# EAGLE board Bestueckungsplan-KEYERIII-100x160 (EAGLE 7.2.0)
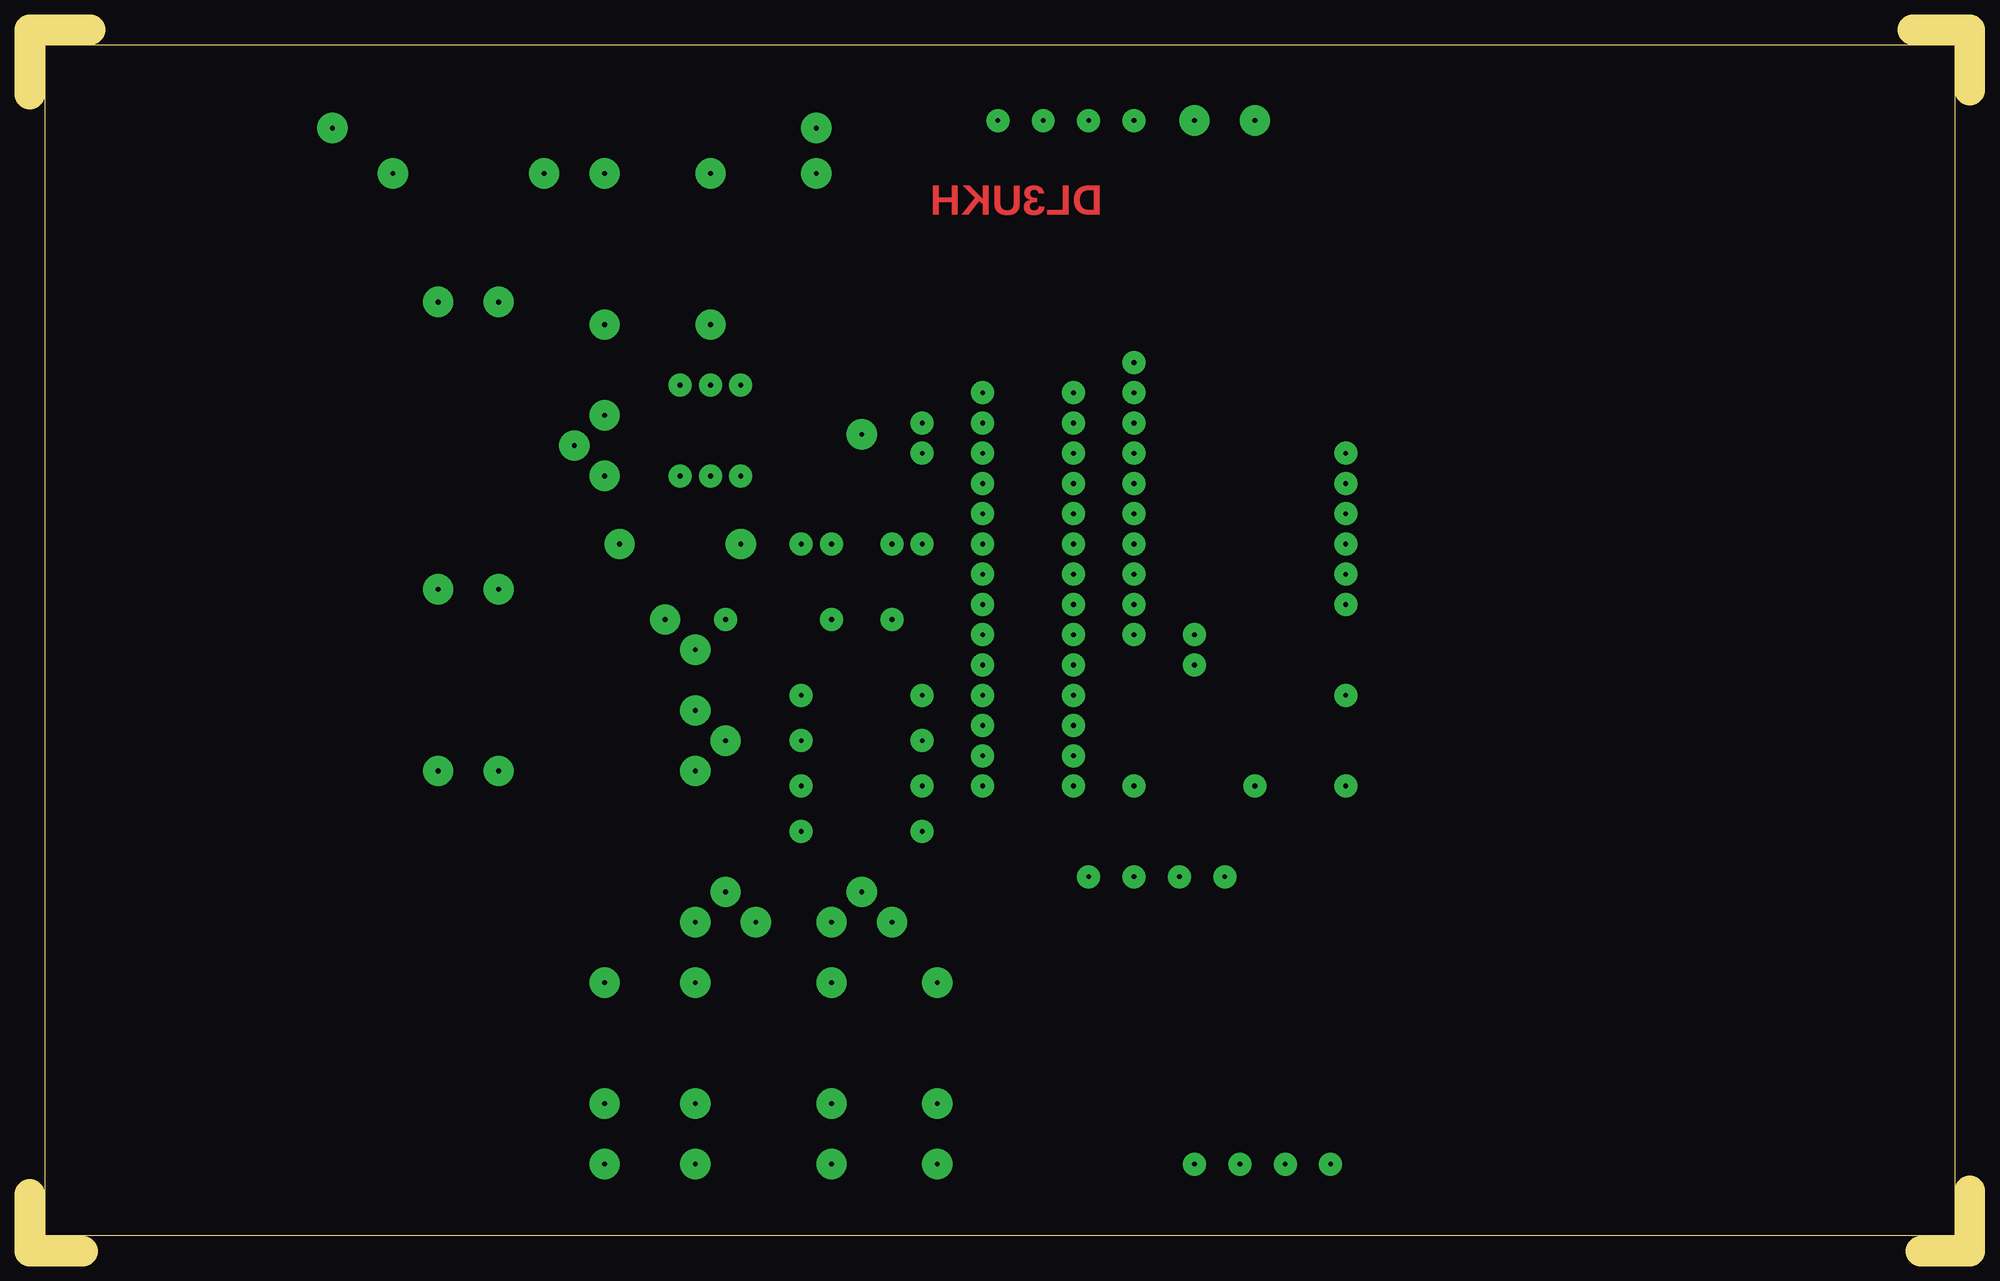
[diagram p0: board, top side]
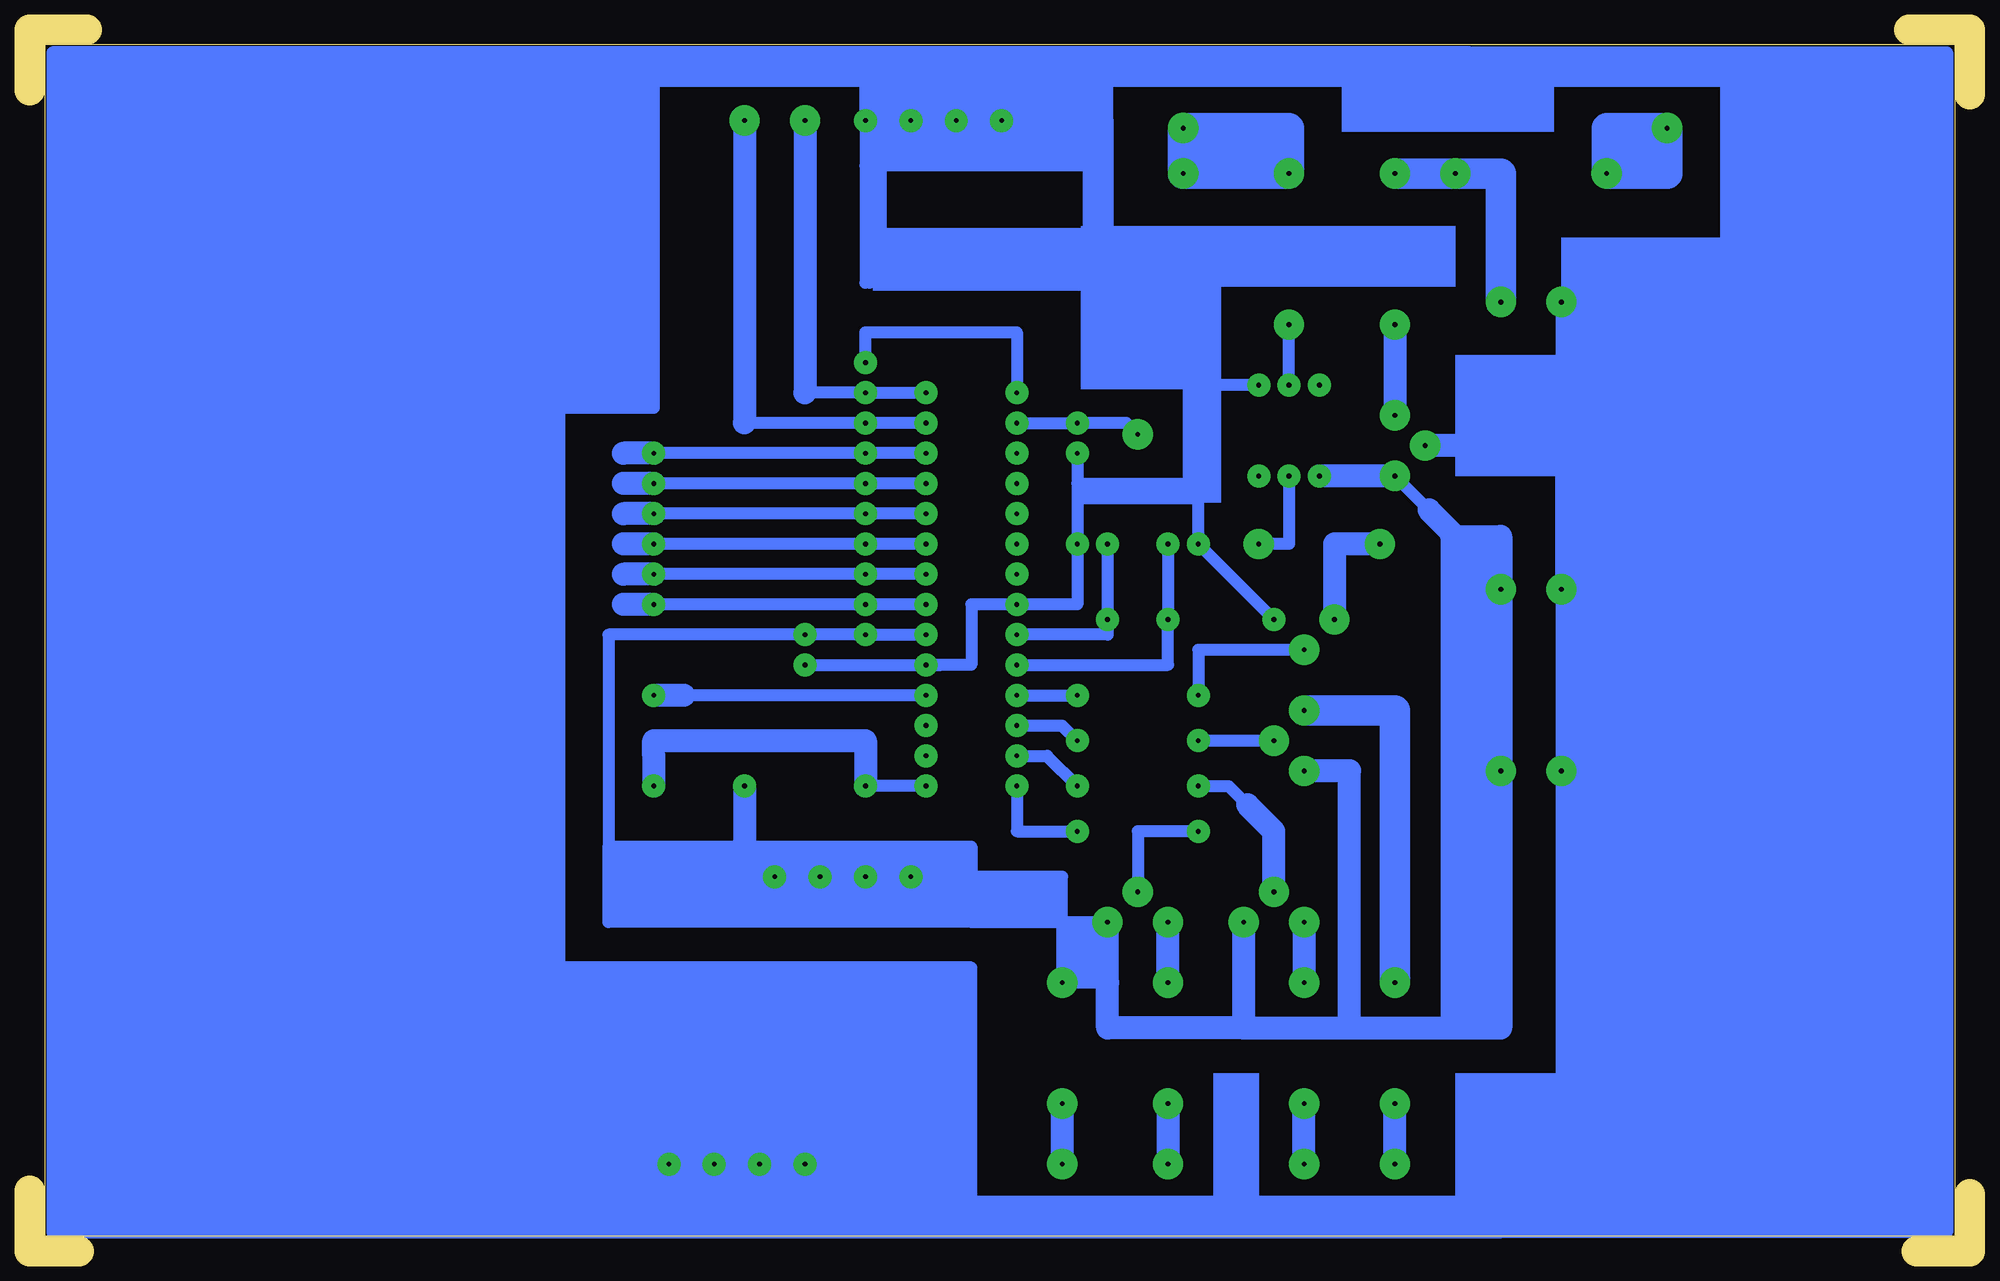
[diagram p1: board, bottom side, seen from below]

Size 162.88 x 102.55 mm. Coordinates in mm from the lower left corner, seen from the top.
Outline: 0,97.16 0,102.23
Outline: 0,102.55 5.08,102.55
Outline: 0,4.76 0,0 4.45,0
Outline: 162.88,97.47 162.88,102.55 158.12,102.55
Outline: 158.75,0 162.88,0
Outline: 162.88,5.08 162.88,0.32
Outline: 1.27,101.28 1.27,1.27 161.61,1.27 161.61,101.28 1.27,101.28
Copper layers (1*16): Top 0.035mm / dielectric 1.5mm / Bottom 0.035mm
Design rules "default": minimum track width 10mil, minimum drill 24mil, track to track 8mil, track to pad 8mil, pad to pad 8mil, via to via 8mil, smd to smd 8mil, copper to edge 40mil, drill to drill 8mil, minimum pad ring 10mil, minimum via ring 8mil, stop-mask expansion 4mil, vias tented up to drill 0mil, thermal gap 10mil

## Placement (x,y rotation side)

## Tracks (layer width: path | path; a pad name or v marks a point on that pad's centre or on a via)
S$1  (via drill 0.4 pad 1.93)
  Bottom 1.016: v80.01,39.05 80.01,35.24 v74.93,35.24
S$2  (via drill 0.4 pad 1.93)
  other vias: 80.01,41.59
S$3  (via drill 0.4 pad 1.93)
  Bottom 1.016: v80.01,44.13 76.2,44.13 v74.93,42.86
S$4  (via drill 0.4 pad 1.93)
  Bottom 1.016: v80.01,46.67 v74.93,46.67
S$5  (via drill 0.4 pad 1.93, 0.4 pad 2.54)
  Bottom 1.016: v55.88,50.48 64.77,50.48 v64.77,46.67
S$6  (via drill 0.4 pad 1.93, 0.4 pad 2.54)
  Bottom 1.016: v64.77,42.86 v58.42,42.86
S$7  (via drill 0.4 pad 1.93)
  Bottom 1.016: 79.69,41.59 77.47,41.59 v74.93,39.05
S$8  (via drill 0.4 pad 1.93)
  other vias: 80.01,56.83
S$9  (via drill 0.4 pad 1.93)
  other vias: 80.01,59.37
S$10  (via drill 0.4 pad 1.93)
  other vias: 80.01,61.91
S$11  (via drill 0.4 pad 1.93)
  other vias: 80.01,64.45
S$12  (via drill 0.4 pad 1.93)
  other vias: 80.01,66.99
S$13  (via drill 0.4 pad 1.93)
  other vias: 88.9,31.43
S$14  (via drill 0.4 pad 2.54)
  Bottom 1.016: v48.26,22.54 48.26,40.01 | 53.66,45.4 v55.88,45.4
  Bottom 2.54: v48.26,22.54 48.26,45.4 v55.88,45.4
S$15  (via drill 0.4 pad 1.93)
  Bottom 1.016: v87.63,39.05 92.71,39.05 | 110.49,41.59 v110.49,39.05
  Bottom 1.93: 110.49,41.59 110.49,42.86 92.71,42.86 92.71,39.05
S$16  (via drill 0.4 pad 1.93)
  other vias: 87.63,41.59
S$17  (via drill 0.4 pad 1.93)
  other vias: 87.63,44.13
S$18  (via drill 0.4 pad 1.93)
  Bottom 1.016: v87.63,46.67 110.49,46.67
S$19  (via drill 0.4 pad 1.93)
  Bottom 1.016: v72.39,59.37 v72.39,53.02 72.39,51.75 v80.01,51.75
S$20  (via drill 0.4 pad 1.93)
  other vias: 110.49,46.67
S$21  (via drill 0.4 pad 1.93)
  other vias: 87.63,54.29
S$22  (via drill 0.4 pad 1.93)
  other vias: 87.63,56.83
S$23  (via drill 0.4 pad 1.93)
  other vias: 87.63,59.37
S$24  (via drill 0.4 pad 1.93)
  other vias: 87.63,61.91
S$25  (via drill 0.4 pad 1.93)
  other vias: 87.63,64.45
S$26  (via drill 0.4 pad 1.93)
  other vias: 87.63,66.99
S$27  (via drill 0.4 pad 1.93)
  other vias: 87.63,69.53
S$28  (via drill 0.4 pad 1.93)
  Bottom 1.016: v80.01,49.21 67.31,49.21 v67.31,53.02 v67.31,59.37
S$29  (via drill 0.4 pad 1.93)
  other vias: 97.79,7.3
S$30  (via drill 0.4 pad 1.93)
  other vias: 96.52,31.43
S$31  (via drill 0.4 pad 1.93, 0.4 pad 2.54)
  Bottom 1.016: v92.71,69.53 102.87,69.53
  Bottom 1.93: v102.87,94.93 102.87,69.53
S$32  (via drill 0.4 pad 1.93)
  other vias: 92.71,66.99
S$33  (via drill 0.4 pad 1.93)
  other vias: 92.71,64.45
S$34  (via drill 0.4 pad 1.93)
  other vias: 92.71,61.91
S$35  (via drill 0.4 pad 1.93)
  other vias: 92.71,59.37
S$36  (via drill 0.4 pad 1.93)
  other vias: 92.71,56.83
S$37  (via drill 0.4 pad 1.93)
  other vias: 92.71,54.29
S$38  (via drill 0.4 pad 2.54)
  Bottom 1.93: v48.26,7.3 v48.26,12.38
S$39  (via drill 0.4 pad 1.93, 0.4 pad 2.54)
  Bottom 1.016: v64.77,35.24 69.85,35.24 v69.85,30.16
S$40  (via drill 0.4 pad 2.54)
  Bottom 1.016: v66.04,90.49 66.36,90.49
  Bottom 2.54: v57.15,90.49 v66.04,90.49 v66.04,94.3 57.15,94.3 v57.15,90.49
S$41  (via drill 0.4 pad 1.93)
  Bottom 1.93: v110.49,66.99 113.03,66.99 | 110.49,64.45 113.03,64.45 | 110.49,61.91 113.03,61.91 | 110.49,59.37 113.03,59.37 | 110.49,56.83 113.03,56.83 | 110.49,54.29 113.03,54.29 | 107.95,46.67 110.49,46.67 | 110.49,41.59 110.49,39.05
S$42  (via drill 0.4 pad 1.93)
  other vias: 110.49,64.45
S$43  (via drill 0.4 pad 1.93)
  other vias: 110.49,61.91
S$44  (via drill 0.4 pad 1.93)
  other vias: 110.49,59.37
S$45  (via drill 0.4 pad 1.93)
  other vias: 110.49,56.83
S$46  (via drill 0.4 pad 1.93)
  other vias: 110.49,54.29
S$47  (via drill 0.4 pad 1.93)
  other vias: 74.93,59.37
S$48  (via drill 0.4 pad 2.54)
  Bottom 1.93: v67.31,22.54 v67.31,27.62
S$49  (via drill 0.4 pad 1.93)
  other vias: 101.6,7.3
S$50  (via drill 0.4 pad 1.93)
  other vias: 100.33,31.43
S$51  (via drill 0.4 pad 1.93, 0.4 pad 2.54)
  Bottom 1.016: v87.63,72.07 v92.71,72.07 97.79,72.07 | 87.63,69.53 v92.71,69.53 | 87.63,66.99 110.49,66.99 | 87.63,64.45 110.49,64.45 | 87.63,61.91 110.49,61.91 | 87.63,59.37 110.49,59.37 | 87.63,56.83 110.49,56.83 | 87.63,54.29 110.49,54.29
  Bottom 1.93: v97.79,94.93 97.79,72.07
S$52  (via drill 0.4 pad 1.93)
  other vias: 105.41,7.3
S$53  (via drill 0.4 pad 2.54)
  Bottom 1.93: v55.88,27.62 v55.88,22.54
S$56  (via drill 0.4 pad 1.93)
  other vias: 92.71,39.05
S$57  (via drill 0.4 pad 2.54)
  Bottom 1.93: v76.2,12.38 v76.2,7.3
S$58  (via drill 0.4 pad 1.93)
  other vias: 88.9,94.93
S$59  (via drill 0.4 pad 2.54)
  Bottom 1.93: v67.31,12.38 v67.31,7.3
S$60  (via drill 0.4 pad 1.93, 0.4 pad 2.54)
  Bottom 1.016: v57.15,72.71 v57.15,77.79
S$61  (via drill 0.4 pad 2.54)
  Bottom 1.93: v55.88,7.3 v55.88,12.38
S$62  (via drill 0.4 pad 1.93)
  other vias: 109.22,7.3
S$63
  Bottom 1.016: 92.71,94.61 92.71,91.12 | 92.71,91.12 92.71,81.28 | 72.71,91.12 73.98,91.12 | 73.98,91.12 91.44,91.12 | 91.44,91.12 92.71,91.12 | 72.71,85.41 73.98,85.41 | 73.98,85.41 91.44,85.41 | 91.44,85.41 92.39,85.41 92.39,81.28 | 73.98,91.12 73.98,85.41 | 91.44,91.12 91.44,85.41
S$64  (via drill 0.4 pad 2.54)
  Bottom 1.93: v48.26,77.79 v48.26,70.17
S$65  (via drill 0.4 pad 1.93)
  other vias: 92.71,31.43
S$66
  Bottom 1.93: 31.75,67.63 46.04,67.63
S$67  (via drill 0.4 pad 2.54)
  Bottom 1.93: v48.26,90.49 v43.18,90.49 39.37,90.49
  Bottom 2.54: v39.37,79.69 39.37,90.49 v48.26,90.49
S$68  (via drill 0.4 pad 2.54)
  Bottom 2.54: v25.4,94.3 30.48,94.3 v30.48,90.49 25.4,90.49 v25.4,94.3
S$69  (via drill 0.4 pad 1.93, 0.4 pad 2.54)
  Bottom 1.016: v80.01,69.53 v74.93,69.53 70.8,69.53 v69.85,68.58
S$70  (via drill 0.4 pad 1.93, 0.4 pad 2.54)
  Bottom 1.016: 60.96,19.37 60.96,18.73 | v87.63,51.75 v92.71,51.75 v97.79,51.75 114.3,51.75 114.3,33.97 | 114.3,33.97 102.87,33.97 | 102.87,33.97 83.82,33.97 83.82,31.43 | 102.87,34.29 102.87,33.97 | 83.82,31.43 83.82,27.62 | 83.82,27.62 76.2,27.62 | 76.2,27.62 v72.39,27.62 | 76.2,27.62 v76.2,22.54 72.39,22.54 | 83.82,27.62 114.3,27.62 114.3,33.97 | 76.2,27.62 76.2,31.43 83.82,31.43 | v48.26,65.09 45.4,62.23
  Bottom 1.93: v48.26,65.09 v54.61,65.09 | v72.39,27.62 72.39,22.54 72.39,18.73 60.96,18.73 52.07,18.73 | 52.07,18.73 52.07,40.32 v55.88,40.32 | 52.07,18.73 39.37,18.73 v39.37,40.32 v39.37,55.56 39.37,60.01 43.18,60.01 | v102.87,39.05 102.87,34.29 | v60.96,27.62 60.96,19.37 | 43.18,60.01 45.4,62.23 | 43.18,60.01 43.5,60.01 43.5,19.05
S$71
  Bottom 1.93: 73.02,81.6 64.14,72.71
S$72  (via drill 0.4 pad 1.93)
  Bottom 1.016: v80.01,72.07 80.01,77.15 82.87,77.15 90.17,77.15 92.71,77.15 v92.71,74.61
S$73  (via drill 0.4 pad 2.54)
  Bottom 1.016: 34.29,67.63 v34.29,55.56 v34.29,40.32 34.29,2.22 | v45.72,67.63 34.29,67.63 | v34.29,79.69 34.29,67.63
S$74  (via drill 0.4 pad 1.93)
  Bottom 1.016: 88.9,94.93 v92.71,94.93 92.71,99.06 | 88.9,94.93 v85.09,94.93 | 41.91,100.65 88.9,100.65 | 88.9,100.65 88.9,94.93 | 88.9,100.65 118.43,100.65 | 118.43,100.65 118.43,23.81 | 118.43,23.81 118.43,1.59 | 118.43,1.59 39.37,1.59 | 39.37,1.59 18.1,4.13 83.82,4.13 83.82,23.81 118.43,23.81 | 41.91,100.65 2.22,99.38 72.39,99.38 | 41.91,100.65 1.91,100.65 1.91,1.91 | 14.92,1.91 1.91,1.91 | 1.91,1.91 1.91,1.59 39.37,1.59 | 118.43,100.65 160.97,100.65 160.97,1.59 118.43,1.59 | 85.09,95.25 v85.09,94.93 | 72.71,80.96 72.39,80.96 | 72.39,80.96 64.77,73.34 64.77,64.45 | v87.63,49.21 86.36,49.21 | v87.63,49.21 83.82,49.21 83.82,54.29 v80.01,54.29 74.93,54.29 74.93,64.45 | v97.79,49.21 v87.63,49.21 | v74.93,66.99 74.93,64.45 | 74.93,64.45 64.77,64.45 | 64.77,63.18 v64.77,59.37 v58.42,53.02 | 64.77,63.18 64.77,64.45 | v85.09,94.93 v81.28,94.93 72.39,94.93 | 72.39,94.93 72.39,80.96 | 72.39,99.38 110.49,99.38 | 110.49,99.38 122.24,98.74 | 72.39,94.93 72.39,99.38 | 110.49,99.38 110.49,70.8 118.74,70.8 | 64.77,63.18 74.61,63.18
S$75  (via drill 0.4 pad 1.93)
  other vias: 54.61,72.71
S$76  (via drill 0.4 pad 1.93)
  Bottom 1.016: v59.69,72.71 64.45,72.71
S$77  (via drill 0.4 pad 1.93)
  other vias: 59.69,65.09
S$78  (via drill 0.4 pad 1.93, 0.4 pad 2.54)
  Bottom 1.016: v57.15,65.09 57.15,59.37 v59.69,59.37
S$79  (via drill 0.4 pad 1.93, 0.4 pad 2.54)
  Bottom 1.016: v64.77,39.05 62.23,39.05 60.64,37.47 | v58.42,30.16 58.42,35.24
  Bottom 1.93: 58.42,29.84 58.42,35.24 60.64,37.47
S$80  (via drill 0.4 pad 2.54)
  Bottom 1.016: v53.34,53.02 53.34,52.7
  Bottom 1.93: v49.53,59.37 53.34,59.37 v53.34,53.02
(copper drawn outside any net)
  shapes: Bottom area x32

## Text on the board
Top: DL3UKH
Vias: Auf Bestückungsseite gesehen !
Dimension: Cevausit 1,5mm dick | alles mit 0,8mm vorgebohrt
tOrigins: CW-Ausg. | +12Volt | 78L05 | Duo-LED a + b | in Fassung | so einbauen | Masse | Punkt | Paddle | Strich | Masse | gn | Stehwelle | 1N4148 | grün | rt | A | 220µ | 220µ | ACHTUNG: | Kurzschluß-Gefahr | Ausg. | Eing. | 470µ/25V | Beine kommen zusammen | rot | + | Masse | Masse | 6 | 4 | 28 | 4N33 und | 1 | µA78L05 | PIC16F876-20SP | Eing. | BC547+BC557 | Poti | 47n | 9x10K | 4N33 | 5K | Text1 | Text1 | 1 | Die Aussparung | 1 | 3 | Text2 | Links oben ist | muß mit dem | Text3 | immer PIN 1 | Bauelement | 470 | BC547c | Text4 | + | 15p | 15p | und dem Bestück- | 8,0MHZ | Text5 | ungsplan | Text6 | überein stimmen. | 470µ/25V | K | 47n | + | K | K | E | 18K | Mithörton | BC557c | B | + | 18K | 14 | 15 | 10K | Programmier | 18K | 1N4148 | 470µ/25V | +5Volt | 18K | A | BC557c | BC557c | K | K | 470 | 270 | 270 | 470 | Widerstandsnetzwerk 9x10K | LEDa gn Programmieren | LEDb rt CW-Ende | LEDb gn CW-Normal | LEDa rt Netzkontrolle | Der Punkt auf dem Bauelement muß | Masse | mit dem Punkt auf dem Bestückungs- | plan hier übereinstimmen, so daß das | Bauelement richtig herum eingelötet | wird.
